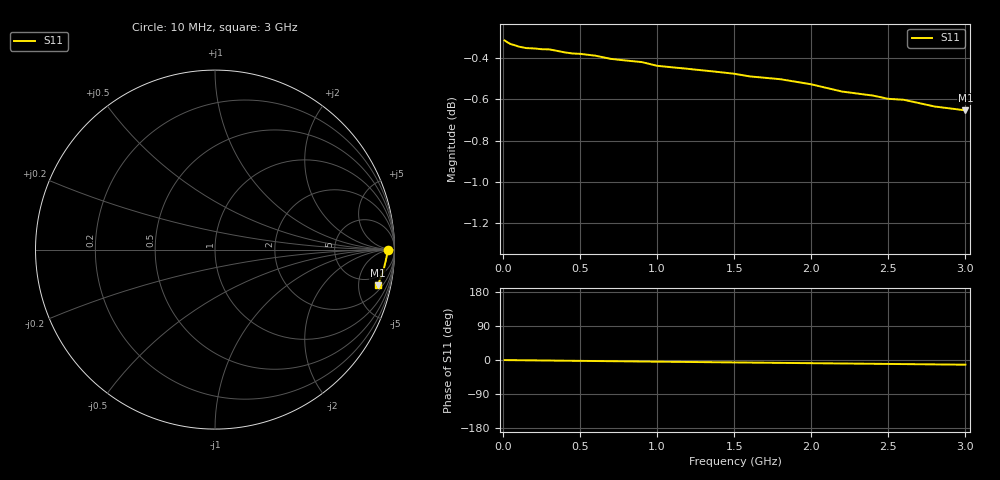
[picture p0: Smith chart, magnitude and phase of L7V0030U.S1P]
! SIEMENS Small Signal Semiconductors
! BAR14-1
! Si PIN Diode in SOT23
! IF = 0.03 mA
! S-Parameters:  July  1992
# GHz  S  MA  R  50
!  f  S11
! GHz  MAG  ANG
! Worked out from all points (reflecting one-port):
!   31 points, 10 MHz to 3 GHz, reference 50 ohm
!   lowest |S11| = -0.7 dB at 3 GHz (marker M1), VSWR 26.62, Z = 144 - j411 ohm
!   phase of S11 starts at -0 deg and turns -12 deg over the sweep
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0.01  0.9646 -0.2
0.05  0.9626 -0.4
0.06  0.9624 -0.4
0.1  0.9613 -0.6
0.15  0.9605 -0.8
0.2  0.9603 -1.0
0.25  0.9599 -1.2
0.3  0.9598 -1.4
0.35  0.959 -1.7
0.4  0.9582 -1.9
0.45  0.9576 -2.1
0.5  0.9574 -2.3
0.6  0.9564 -2.7
0.7  0.9547 -3.1
0.8  0.9538 -3.5
0.9  0.953 -4.0
1  0.951 -4.4
1.2  0.9494 -5.2
1.5  0.9468 -6.4
1.6  0.9454 -6.8
1.8  0.9439 -7.6
2  0.9412 -8.4
2.2  0.9374 -9.2
2.4  0.9353 -10.0
2.5  0.9336 -10.4
2.6  0.9331 -10.8
2.8  0.9296 -11.6
3  0.9276 -12.4
